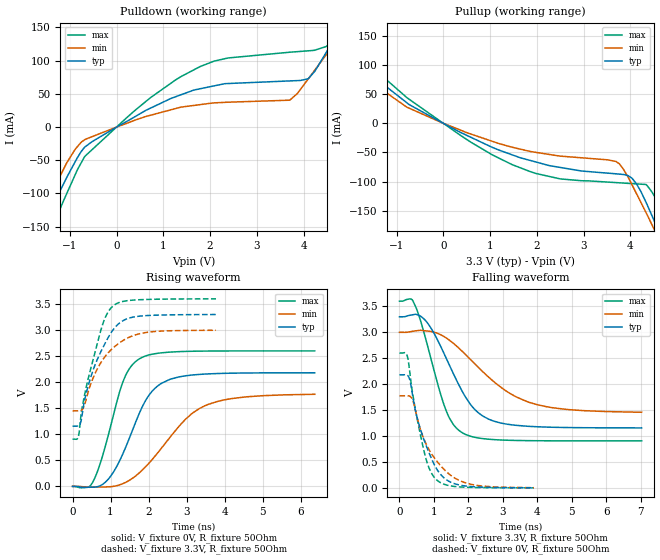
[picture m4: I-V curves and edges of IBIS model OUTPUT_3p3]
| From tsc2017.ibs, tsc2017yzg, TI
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|   output_3p3 Model
[Model]   OUTPUT_3p3
Model_type   Output
Polarity   Non-Inverting
Enable   Active-Low
Vmeas = 1.65
Vref = 1.65
Cref = 15pF
Rref = 50
|   typ   min   max
|   (nom PVT)   (Fast PVT)   (slow PVT)
|Average
C_comp   1.195e-11   1.117e-11   1.308e-11
|ON state : BUFFER OUTPUT TURNED HIGH
|C_comp   1.109e-11   9.866e-12   1.267e-11
|OFF state: BUFFER OUTPUT TURNED LOW
|C_comp   1.281e-11   1.247e-11   1.348e-11
|C_comp from frequency method(F=3.4MHz)
| Where nom  PVT is Nominal Process, 3.3V, 25C
|   Fast PVT is Strong Process,  3.6V, -40C
|   Slow PVT is Weak Process,   3V, 85C
[Voltage Range]   3.3   3   3.6
|Ambient Temperature   25   85   -40
|Junction Temperature
[Temperature Range]   25   85   -40
[Pullup Reference]   3.3   3   3.6
[Pulldown Reference]   0   0   0
[Power Clamp Reference]   3.3   3   3.6
[GND Clamp Reference]   0   0   0
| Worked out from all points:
|   slope of the pulldown table from 0 to 0.495 V, typ, clamps not added: 25 ohm
|   slope of the pullup table from 0 to 0.495 V, typ, clamps not added: 24.2 ohm
|   falling waveform, V_fixture 3.3V, R_fixture 50Ohm: 20-80 % time 999ps typ, 1.62ns min, 699ps max; typ from 3.3 V to 1.16 V
|   rising waveform, V_fixture 0V, R_fixture 50Ohm: 20-80 % time 806ps typ, 1.28ns min, 605ps max; typ from 0 V to 2.18 V
|   rising waveform, V_fixture 3.3V, R_fixture 50Ohm: 20-80 % time 650ps typ, 724ps min, 534ps max; typ from 1.16 V to 3.3 V
|   falling waveform, V_fixture 0V, R_fixture 50Ohm: 20-80 % time 628ps typ, 801ps min, 460ps max; typ from 2.18 V to 0.002 V
[Pulldown]
|   Voltage   I(typ)   I(min)   I(max)
-3.3V     -497.6mA   -417.5mA   -634.3mA
-1.766V   -192.7mA   -160.7mA   -234.4mA
-1.576V   -156mA     -129.6mA   -188.6mA
-1.398V   -124.3mA   -100.7mA   -154.7mA
-676.5mV  -29.89mA   -18.87mA   -44.07mA
1.79V     57.71mA    33.8mA     91.17mA
3.702V    69.47mA    40.47mA    112.7mA
4.105V    73.02mA    72.9mA     114.8mA
4.494V    113.3mA    109.6mA    121.7mA
4.778V    146.4mA    129.1mA    159.2mA
5.135V    175.5mA    149.1mA    210.4mA
6.6V      238.5mA    201.1mA    300.8mA
[Pullup]
|   Voltage   I(typ)   I(min)   I(max)
-3.3V     154.6mA    145.5mA    165.1mA
-1.972V   111.4mA    101.7mA    124.6mA
-780mV    35.27mA    27.69mA    44.12mA
595.2mV   -24.22mA   -18.55mA   -32.67mA
1.474V    -54.11mA   -41.05mA   -70.96mA
2.5V      -75.68mA   -56.23mA   -95.36mA
3.693V    -86.64mA   -65.41mA   -101.7mA
4.039V    -94.65mA   -106.1mA   -103.5mA
4.336V    -135.6mA   -153.4mA   -105mA
4.528V    -170.6mA   -185.2mA   -126.9mA
4.811V    -224.4mA   -233mA     -180.1mA
6.6V      -575.4mA   -540.3mA   -637.9mA
[Ramp]
R_load = 50
|   typ   min   max
dV/dt_r   1.30863/8.06118e-10   1.06573/1.29078e-09   1.56046/6.04502e-10
dV/dt_f   1.2862/9.99448e-10   0.92999/1.641e-09   1.61614/6.97773e-10
[Falling Waveform]
V_fixture = 3.3V
V_fixture_min = 3V
V_fixture_max = 3.6V
R_fixture = 50Ohm
|   Time   V(typ)   V(min)   V(max)
0s        3.3V       3V         3.6V
400ps     3.341V     3.022V     3.593V
800ps     3.192V     3.026V     2.78V
1.35ns    2.511V     2.895V     1.498V
1.575ns   2.188V     2.782V     1.213V
1.85ns    1.828V     2.615V     1.053V
2.175ns   1.52V      2.399V     977.1mV
2.575ns   1.33V      2.143V     939.4mV
3.75ns    1.187V     1.653V     911.1mV
7.025ns   1.157V     1.459V     906.5mV
[Rising Waveform]
V_fixture = 0V
V_fixture_min = 0V
V_fixture_max = 0V
R_fixture = 50Ohm
|   Time   V(typ)   V(min)   V(max)
0s        864.9pV    3.026nV    624.8pV
400ps     -16.18mV   -14.7mV    -17.48mV
550ps     -14.96mV   -13.19mV   106.6mV
925ps     126.5mV    -8.929mV   939.8mV
1.325ns   627.8mV    52.95mV    2.005V
1.8ns     1.474V     288.9mV    2.465V
2.35ns    1.982V     743.5mV    2.565V
2.975ns   2.123V     1.29V      2.591V
3.475ns   2.156V     1.545V     2.597V
6.375ns   2.181V     1.768V     2.601V
[Rising Waveform]
V_fixture = 3.3V
V_fixture_min = 3V
V_fixture_max = 3.6V
R_fixture = 50Ohm
|   Time   V(typ)   V(min)   V(max)
0s        1.156V     1.45V      906.4mV
150ps     1.16V      1.45V      943.8mV
225ps     1.258V     1.459V     1.388V
325ps     1.683V     1.584V     1.787V
475ps     2.087V     1.957V     2.25V
675ps     2.477V     2.287V     2.808V
850ps     2.737V     2.487V     3.223V
1.05ns    2.989V     2.647V     3.452V
1.65ns    3.257V     2.907V     3.579V
3.775ns   3.299V     2.997V     3.6V
[Falling Waveform]
|Gnd
V_fixture = 0V
V_fixture_min = 0V
V_fixture_max = 0V
R_fixture = 50Ohm
|   Time   V(typ)   V(min)   V(max)
0s        2.181V     1.776V     2.601V
225ps     2.176V     1.776V     2.549V
300ps     2.088V     1.768V     2.233V
375ps     1.812V     1.709V     1.853V
700ps     951.2mV    959.7mV    747.3mV
850ps     690.9mV    748.3mV    398.7mV
1.05ns    400.3mV    544.4mV    174.2mV
1.425ns   131.4mV    275.5mV    45.97mV
2ns       29.88mV    82.33mV    10.88mV
3.9ns     1.951mV    4.286mV    914.1uV
